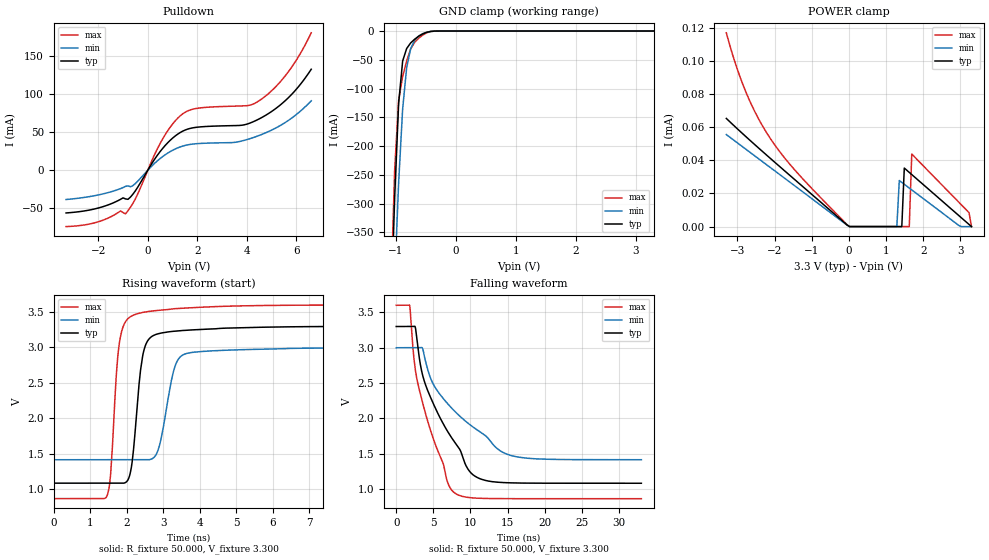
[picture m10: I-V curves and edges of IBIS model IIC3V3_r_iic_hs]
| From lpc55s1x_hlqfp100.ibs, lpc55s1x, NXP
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|   Model IIC3V3_r_iic_hs
[Model] IIC3V3_r_iic_hs
Model_type I/O_open_drain
Polarity   Non-Inverting
Enable   Active-Low
Vinl =  0.990V
Vinh =  2.310V
Vmeas =  1.650V
Cref =  0.0F
Rref =  100.000
Vref =  3.3V
C_comp   2.333pF   2.290pF   2.366pF
C_comp_pulldown   1.605pF   1.543pF   1.655pF
C_comp_power_clamp   0.444pF   0.380pF   0.497pF
[Model Spec]
Vinh   2.310V   2.100V   2.520V
Vinl   0.990V   0.900V   1.080V
Vmeas   1.650V   1.500V   1.800V
Vref   3.3V   3.0V   3.6V
Cref   0.0F   0.0F   0.0F
Rref   100.000   100.000   100.000
[Temperature Range]   25.000   0.125k   -40.000
[Voltage Range]   3.300V   3.000V   3.600V
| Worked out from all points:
|   slope of the pulldown table from 0 to 0.495 V, typ, clamps not added: 20.4 ohm
|   GND clamp passes 1 mA (typ) near -0.43 V on its own axis
|   rising waveform, R_fixture 50.000, V_fixture 3.300: 20-80 % time 249ps typ, 344ps min, 210ps max; typ from 1.08 V to 3.3 V
|   falling waveform, R_fixture 50.000, V_fixture 3.300: 20-80 % time 5.6ns typ, 8ns min, 3.93ns max; typ from 3.3 V to 1.08 V
[Pulldown]
|Voltage   I(typ)   I(min)   I(max)
-3.3V     -56mA      -38.4mA    -73.87mA
-2.1V     -50.37mA   -33.07mA   -68.52mA
-1.1V     -38.15mA   -24.11mA   -53.37mA
-900mV    -37.61mA   -21.16mA   -57.18mA
-500mV    -26.92mA   -17.4mA    -37.43mA
500mV     24.51mA    15.34mA    35.14mA
1.2V      47.07mA    29.16mA    67.89mA
1.9V      55.94mA    34.55mA    80.54mA
3.8V      58.93mA    38.34mA    84.23mA
4.5V      67.27mA    45.57mA    91.11mA
5.6V      92.6mA     63.56mA    125.7mA
6.6V      132.3mA    90.95mA    180mA
[GND_clamp]
|Voltage   I(typ)   I(min)   I(max)
-3.3V     -10.05A    -9.18A     -11.33A
-1.089V   -516.5mA   -633.7mA   -475mA
-1.022V   -291.9mA   -436.3mA   -243.2mA
-955mV    -126mA     -264mA     -120.7mA
-888mV    -52.17mA   -135.6mA   -79.12mA
-821mV    -30.44mA   -63.69mA   -52.12mA
-754mV    -20.67mA   -30.69mA   -31.05mA
-687mV    -14.19mA   -15.97mA   -19.65mA
-553mV    -5.021mA   -4.512mA   -7.044mA
-419mV    -659.6uA   -714.3uA   -896.4uA
-285mV    -20.38uA   -37.42uA   -22.84uA
3.3V      0A         0A         0A
[POWER_clamp]
|Voltage   I(typ)   I(min)   I(max)
-3.3V     65.36uA    55.62uA    117.1uA
-2.797V   54.84uA    47.15uA    82.63uA
-2.194V   42.78uA    37.02uA    55.95uA
-50mV     976.9nA    858.9nA    1.15uA
1.29V     0A         0A         0A
1.357V    0A         27.85uA    0A
1.424V    0A         26.71uA    0A
1.491V    35.37uA    25.58uA    0A
1.625V    32.75uA    23.31uA    0A
1.692V    31.44uA    22.17uA    43.84uA
3.233V    1.309uA    0A         8.433uA
3.3V      0A         0A         0A
[Ramp]
| variable   typ   min   max
dV/dt_r   1.329/0.249n   0.951/0.343n   1.640/0.210n
dV/dt_f   1.329/5.604n   0.950/7.993n   1.640/3.926n
R_load = 50.000
[Rising Waveform]
R_fixture= 50.000
V_fixture= 3.300
V_fixture_min= 3.000
V_fixture_max= 3.600
|time   V(typ)   V(min)   V(max)
0s        1.085V     1.415V     866.6mV
1.471ns   1.085V     1.415V     921.3mV
1.572ns   1.085V     1.415V     1.3V
1.772ns   1.085V     1.415V     2.959V
2.016ns   1.117V     1.415V     3.397V
2.511ns   3.026V     1.414V     3.501V
2.876ns   3.195V     1.576V     3.524V
3.367ns   3.232V     2.789V     3.549V
3.911ns   3.251V     2.936V     3.564V
33ns      3.3V       3V         3.6V
[Falling Waveform]
R_fixture= 50.000
V_fixture= 3.300
V_fixture_min= 3.000
V_fixture_max= 3.600
|time   V(typ)   V(min)   V(max)
0s        3.3V       3V         3.6V
1.807ns   3.3V       3V         3.599V
2.556ns   3.294V     3V         2.702V
3.016ns   2.928V     3V         2.447V
4.277ns   2.385V     2.678V     1.949V
7.79ns    1.677V     2.111V     954.7mV
9.89ns    1.251V     1.915V     881.8mV
12.19ns   1.12V      1.741V     869.6mV
16.63ns   1.088V     1.451V     866.9mV
33ns      1.085V     1.417V     866.6mV
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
